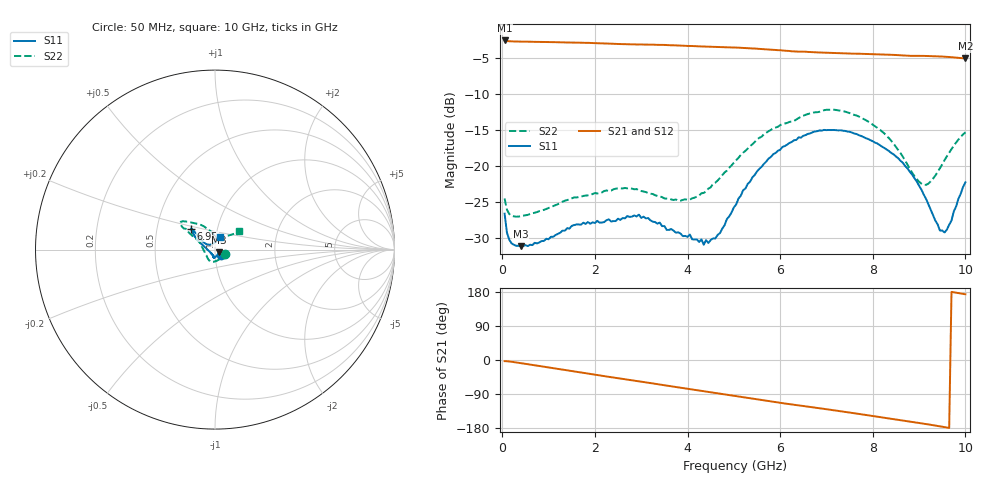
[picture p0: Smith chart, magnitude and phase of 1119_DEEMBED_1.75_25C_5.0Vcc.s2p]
!Hittite Microwave Corp.
!Digital Attenuator/PhaseShifter Rev 1.4.0
!Filename: C:\DATA\DATA\1119_DEEMBED_1.75_25C_5.0Vcc.s2p
!VNA ID: Agilent Technologies,N5224A,MY51441122,A.10.45.03
!Device type:
!2 Port Calibration.
!Temp(C): 25
!Lot Number:
!Serial Number:
!Operator:
!Misc:
!Attenuator:  1.750
# GHZ S DB R 50.0
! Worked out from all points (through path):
!   200 points, 50 MHz to 10 GHz, reference 50 ohm
!   highest |S21| = -2.62 dB at 50 MHz (marker M1); lowest = -5.1 dB at 10 GHz (marker M2)
!   group delay of S21, straight-line fit = 50.9 ps
!   lowest |S11| = -31.1 dB at 400 MHz (marker M3), VSWR 1.06, Z = 52.4 - j1.46 ohm
!   |S11| at or under -10 dB: start of sweep to end of sweep
!   |S22| runs from -27.1 to -12.2 dB; largest |S21 - S12| = 0.0018
!   S11 on the Smith chart (normalised r, x): 50 MHz: 1.07, -0.06; 6.95 GHz: 0.75, +0.18; 10 GHz: 1.05, +0.15
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0.05  -26.63 -39.9  -2.62 -3.0  -2.62 -3.0  -24.53 -26.7
0.1  -29.26 -32.9  -2.71 -3.2  -2.70 -3.2  -26.08 -22.1
0.15  -30.23 -29.4  -2.73 -3.9  -2.73 -3.9  -26.67 -20.2
0.4  -31.14 -30.2  -2.78 -8.3  -2.78 -8.3  -26.98 -24.6
1.75  -27.89 -86.0  -2.94 -33.9  -2.94 -33.9  -24.17 -76.3
2.75  -27.08 -95.8  -3.15 -52.5  -3.16 -52.6  -23.07 -111.3
3.4  -27.87 -105.0  -3.23 -64.6  -3.23 -64.7  -24.24 -134.8
3.85  -29.40 -110.8  -3.33 -73.1  -3.34 -73.2  -24.84 -152.2
4.35  -30.95 -134.0  -3.46 -82.3  -3.47 -82.4  -23.76 178.2
4.7  -29.33 -167.1  -3.54 -88.8  -3.55 -88.9  -21.69 161.4
5.05  -25.37 169.1  -3.61 -95.3  -3.63 -95.3  -19.22 151.8
5.4  -21.61 157.8  -3.73 -102.0  -3.74 -102.0  -17.02 148.6
5.85  -18.39 149.7  -3.91 -110.3  -3.93 -110.4  -14.79 146.0
6.7  -15.35 140.4  -4.24 -124.8  -4.25 -124.8  -12.65 144.0
6.95  -15.02 138.6  -4.31 -129.0  -4.32 -129.0  -12.29 143.0
7.65  -15.59 138.4  -4.46 -141.3  -4.47 -141.4  -13.03 135.8
8.35  -17.96 140.4  -4.60 -154.3  -4.60 -154.3  -16.17 118.9
8.75  -20.37 144.5  -4.74 -161.5  -4.74 -161.5  -19.83 102.5
9.1  -23.98 147.5  -4.76 -168.0  -4.78 -168.0  -22.63 80.8
9.45  -28.97 127.4  -4.83 -175.0  -4.84 -175.0  -20.34 51.4
9.55  -29.24 110.1  -4.87 -177.2  -4.88 -177.2  -19.21 45.9
10  -22.29 68.0  -5.12 173.4  -5.12 173.5  -15.36 37.6
